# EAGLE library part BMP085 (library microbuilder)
BMP085 Digital Pressure Sensor 1.8-3.6V Supply, I2C Interface
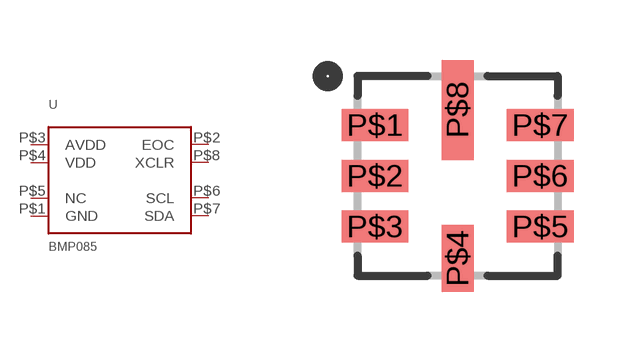
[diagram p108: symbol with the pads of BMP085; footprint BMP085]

Designator prefix U

## BMP085  [BMP085]
P$1  GND
P$2  EOC
P$3  AVDD
P$4  VDD
P$5  NC
P$6  SCL
P$7  SDA
P$8  XCLR

## Footprint BMP085 (pad centres in mm)
smd 1.67 x 0.8: P$1 -2.065,1.27; P$2 -2.065,0; P$3 -2.065,-1.27; P$5 2.065,-1.27; P$6 2.065,0; P$7 2.065,1.27
smd 0.8 x 1.67: P$4 0,-2.065
smd 0.8 x 2.5: P$8 0,1.65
